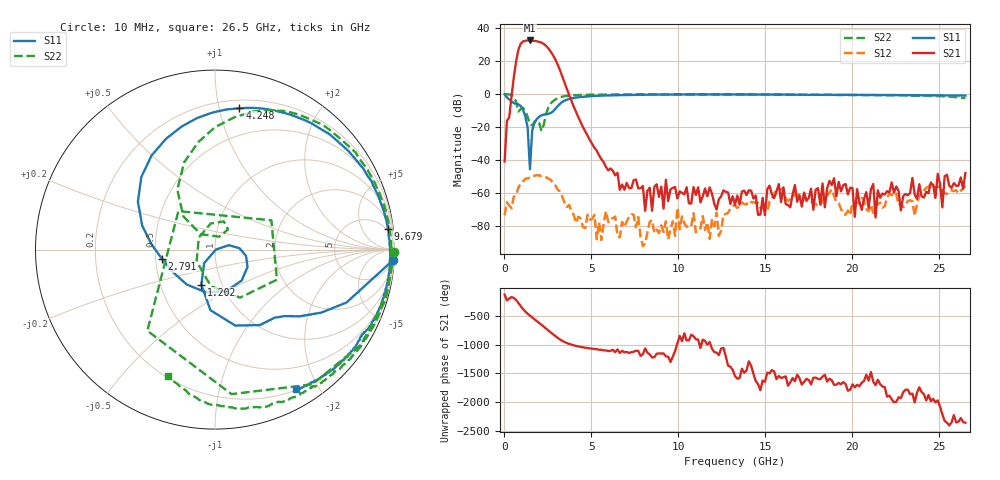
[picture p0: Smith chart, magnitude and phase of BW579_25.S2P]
!Agilent Technologies,N5242A,MY52422126,A.09.90.01
!Agilent N5242A: A.09.90.01
!Date: Wednesday, November 18, 2015 21:25:38
!Correction: S11(Full 2 Port(1,2))
!S21(Full 2 Port(1,2))
!S12(Full 2 Port(1,2))
!S22(Full 2 Port(1,2))
!S2P File: Measurements: S11, S21, S12, S22:
# Hz S  dB  R 50
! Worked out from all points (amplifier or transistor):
!   201 points, 10 MHz to 26.5 GHz, reference 50 ohm
!   highest |S21| = 32.5 dB at 1.467 GHz (marker M1)
!   |S21| within 3 dB of that: 898.2 MHz to 2.365 GHz (1.467 GHz wide, 89.9 % of centre)
!   unconditionally stable (mu >= 1): 11.53 MHz to end of sweep
!   at 4.381 GHz: K = 755.33, MAG = -2.6 dB, |S12| = -75.4 dB
!   at 13.26 GHz: K = 5207.33, MAG = -40.0 dB, |S12| = -67.3 dB
!   at 26.5 GHz: K = 6180.14, MAG = -37.1 dB, |S12| = -55.5 dB
!   S11 on the Smith chart (normalised r, x): 10 MHz: 4, -33; 1.202 GHz: 0.80, -0.33; 2.791 GHz: 0.54, -0.06; 4.248 GHz: 0.26, +1.15; 9.679 GHz: 4, +16; 26.5 GHz: 0.21, -1.71
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1e7  -0.06 -3.5  -40.82 -129.1  -73.49 32.2  -0.00 -0.9
5.398e8  -5.41 -43.6  10.22 171.4  -62.18 -80.4  -1.83 -83.5
8.047e8  -6.21 -59.3  26.99 82.2  -56.62 -140.3  -10.58 133.6
9.3715e8  -7.17 -75.1  30.53 26.1  -54.04 166.7  -9.02 27.5
1.0696e9  -9.41 -94.3  31.90 -23.6  -52.89 119.8  -8.32 -25.9
1.20205e9  -13.53 -111.2  32.29 -65.4  -51.42 81.5  -10.40 -62.5
1.46695e9  -45.53 2.3  32.49 -136.3  -50.69 11.5  -18.31 -147.5
1.73185e9  -17.28 3.2  32.22 159.8  -49.43 -44.1  -16.63 99.4
1.99675e9  -13.74 -28.2  31.63 97.4  -49.31 -97.3  -17.44 57.2
2.26165e9  -12.44 -74.7  30.40 31.4  -49.79 -153.2  -18.64 132.8
2.3941e9  -12.26 -102.1  29.23 -2.5  -50.37 -179.9  -11.87 133.6
2.52655e9  -12.03 -129.1  27.68 -35.8  -51.18 156.2  -8.08 122.1
2.79145e9  -10.45 -170.3  23.57 -100.2  -53.87 105.5  -4.34 98.7
3.1888e9  -5.92 148.1  14.58 170.9  -59.05 35.7  -1.97 74.8
4.2484e9  -1.94 80.2  -14.00 47.8  -74.30 -58.7  -0.56 39.6
4.5133e9  -1.63 71.5  -20.01 31.6  -80.64 -142.0  -0.43 34.7
8.88415e9  -0.31 12.5  -62.29 -73.7  -84.31 -104.2  -0.14 -6.1
9.67885e9  -0.27 6.9  -56.82 -130.5  -77.09 -121.9  -0.14 -10.7
1.3255e10  -0.19 -12.4  -67.04 -107.5  -67.35 -46.1  -0.20 -28.2
1.77583e10  -0.47 -30.5  -70.14 -138.5  -66.71 170.1  -0.41 -48.2
2.212915e10  -0.58 -45.7  -59.57 -87.5  -60.38 -118.2  -0.77 -69.7
2.65e10  -0.93 -60.0  -47.84 161.1  -55.50 -155.1  -2.50 -110.3
